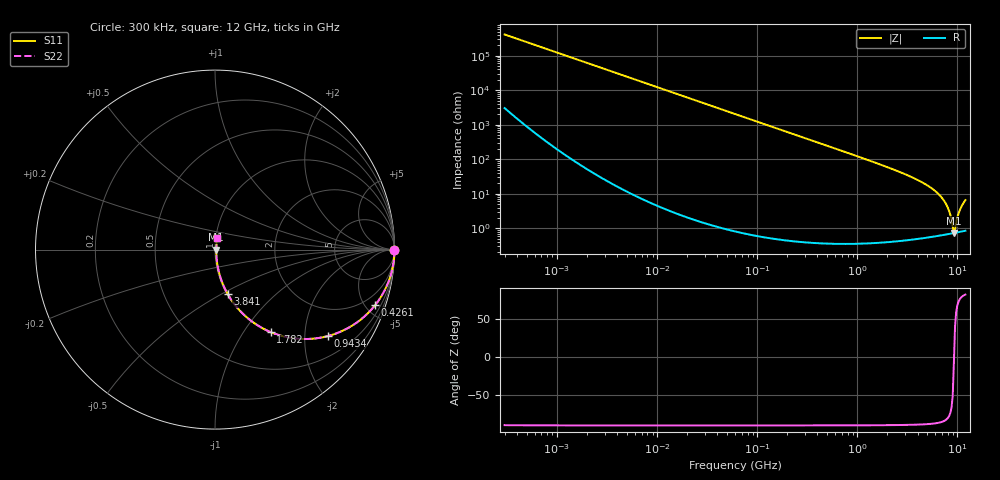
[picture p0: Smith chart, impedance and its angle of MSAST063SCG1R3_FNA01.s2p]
! MSAST063SCG1R3_FNA01  S-PARAMETER MODEL  ( Standard Model )
! Model Generated by TAIYO YUDEN Corporation (http://www.ty-top.com)
! Version 1.0
! TAIYO YUDEN Control No. 241122
! Copyright(c) 2024 TAIYO YUDEN CO.,LTD. All Rights Reserved.
! Product Description (link to TY-COMPAS)
! https://ds.yuden.co.jp/TYCOMPAS/or/detail?pn=MSAST063SCG1R3CFNA01&u=M
! Products Name : Multilayer Ceramic Capacitors
! Characteristics :
!  Capacitance : 1.3 [pF] , Rated Voltage : 25 [V] , TCC : CG / C0G
!  Case Size : 0.6 x 0.3 / 0.024 x 0.012 [mm/inch] , Thickness : 0.3 / 0.012 [mm/inch]
!  (Conditions: Temperature = 25 [degC] , DC Bias Voltage = 0 [V])
! External Node Assignments :
!  1  o---| |---o  2
! GND o---------o GND
! Frequency Range : 0.3MHz  -  12000MHz  [ 401 STEP ]
# MHZ S RI R 50
! Freq[MHz].  S11 Real  S11 Imag  S21 Real  S21 Imag  S12 Real  S12 Imag  S22 Real  S22 Imag
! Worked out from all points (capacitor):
!   401 points, 300 kHz to 12 GHz, reference 50 ohm
!   read as one part in series: C = 1.29 pF near 316.3 kHz
!   lowest |Z| = 736 mohm at 9.207 GHz (marker M1)
!   series resonance near 9.241 GHz, so ESL is about 230 pH
!   S11 on the Smith chart (normalised r, x): 300 kHz: open; 426.1 MHz: 1.01, -5.79; 943.4 MHz: 1.01, -2.59; 1.782 GHz: 1.01, -1.34; 3.841 GHz: 1.01, -0.53; 12 GHz: 1.02, +0.13
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0.3  1 -0.000243  1.84e-06 0.000243  1.84e-06 0.000243  1 -0.000243
1.769972  1 -0.00143  3.36e-06 0.00143  3.36e-06 0.00143  1 -0.00143
10.44266  0.9999 -0.00844  7.44e-05 0.00844  7.44e-05 0.00844  0.9999 -0.00844
60  0.9976 -0.0484  0.00237 0.0484  0.00237 0.0484  0.9976 -0.0484
159.8975  0.9835 -0.1272  0.0165 0.1272  0.0165 0.1272  0.9835 -0.1272
353.9943  0.9238 -0.2648  0.0762 0.2648  0.0762 0.2648  0.9238 -0.2648
426.1204  0.8931 -0.3083  0.1069 0.3083  0.1069 0.3083  0.8931 -0.3083
634.0297  0.7899 -0.4065  0.2101 0.4065  0.2101 0.4065  0.7899 -0.4065
943.3804  0.6269 -0.4823  0.3731 0.4823  0.3731 0.4823  0.6269 -0.4823
1781.601  0.3098 -0.4595  0.6902 0.4595  0.6902 0.4595  0.3098 -0.4595
2088.533  0.2416 -0.4245  0.7584 0.4245  0.7584 0.4245  0.2416 -0.4245
3841.137  0.0703 -0.2467  0.9297 0.2467  0.9297 0.2467  0.0703 -0.2467
5420.343  0.0272 -0.1452  0.9728 0.1452  0.9728 0.1452  0.0272 -0.1452
6879.757  0.0126 -0.0792  0.9874 0.0792  0.9874 0.0792  0.0126 -0.0792
7854.144  0.00857 -0.0437  0.9914 0.0437  0.9914 0.0437  0.00857 -0.0437
8281.503  0.00772 -0.0297  0.9923 0.0297  0.9923 0.0297  0.00772 -0.0297
8966.534  0.00721 -0.00868  0.9928 0.00868  0.9928 0.00868  0.00721 -0.00868
9207.246  0.00724 -0.00096  0.9928 0.00096  0.9928 0.00096  0.00724 -0.00096
9708.23  0.00761 0.0125  0.9924 -0.0125  0.9924 -0.0125  0.00761 0.0125
10236.47  0.00831 0.0249  0.9917 -0.0249  0.9917 -0.0249  0.00831 0.0249
10793.46  0.00933 0.0373  0.9907 -0.0373  0.9907 -0.0373  0.00933 0.0373
12000  0.0125 0.0637  0.9875 -0.0637  0.9875 -0.0637  0.0125 0.0637
